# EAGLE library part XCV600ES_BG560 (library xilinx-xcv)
xcv600es_bg560 edit this description Auto generated by make-symbol-device-package-bsdl.ulp Rev. 26 Source: xcv600es_bg560.bsd
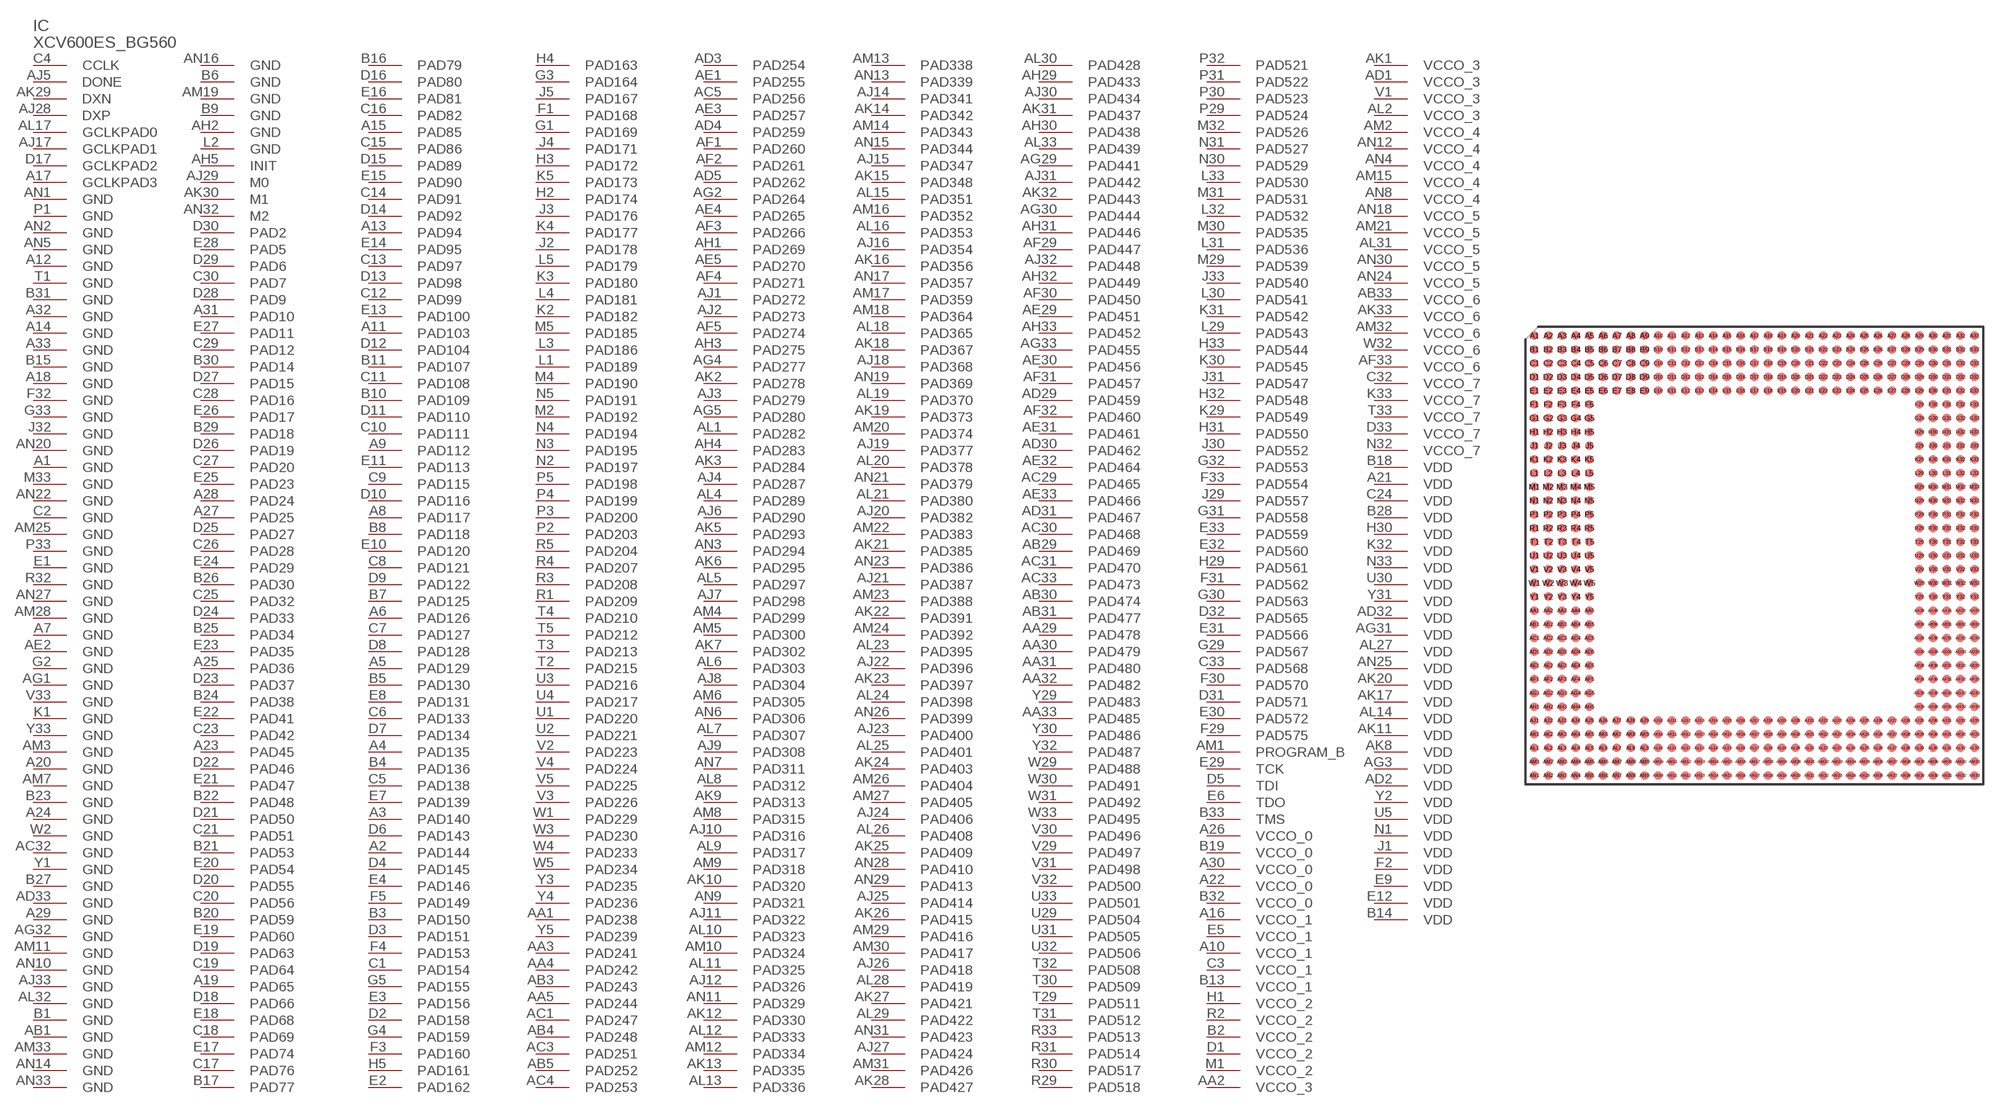
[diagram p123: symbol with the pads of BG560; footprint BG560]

Designator prefix IC

## XCV600ES_BG560 (OC_FARNELL: unknown; OC_NEWARK: unknown)  [BG560]
A1  GND  pwr
A2  PAD144
A3  PAD140
A4  PAD135
A5  PAD129
A6  PAD126
A7  GND  pwr
A8  PAD117
A9  PAD112
A10  VCCO_1  pwr
A11  PAD103
A12  GND  pwr
A13  PAD94
A14  GND  pwr
A15  PAD85
A16  VCCO_1  pwr
A17  GCLKPAD3  in
A18  GND  pwr
A19  PAD65
A20  GND  pwr
A21  VDD  pwr
A22  VCCO_0  pwr
A23  PAD45
A24  GND  pwr
A25  PAD36
A26  VCCO_0  pwr
A27  PAD25
A28  PAD24
A29  GND  pwr
A30  VCCO_0  pwr
A31  PAD10
A32  GND  pwr
A33  GND  pwr
AA1  PAD238
AA2  VCCO_3  pwr
AA3  PAD241
AA4  PAD242
AA5  PAD244
AA29  PAD478
AA30  PAD479
AA31  PAD480
AA32  PAD482
AA33  PAD485
AB1  GND  pwr
AB3  PAD243
AB4  PAD248
AB5  PAD252
AB29  PAD469
AB30  PAD474
AB31  PAD477
AB33  VCCO_6  pwr
AC1  PAD247
AC3  PAD251
AC4  PAD253
AC5  PAD256
AC29  PAD465
AC30  PAD468
AC31  PAD470
AC32  GND  pwr
AC33  PAD473
AD1  VCCO_3  pwr
AD2  VDD  pwr
AD3  PAD254
AD4  PAD259
AD5  PAD262
AD29  PAD459
AD30  PAD462
AD31  PAD467
AD32  VDD  pwr
AD33  GND  pwr
AE1  PAD255
AE2  GND  pwr
AE3  PAD257
AE4  PAD265
AE5  PAD270
AE29  PAD451
AE30  PAD456
AE31  PAD461
AE32  PAD464
AE33  PAD466
AF1  PAD260
AF2  PAD261
AF3  PAD266
AF4  PAD271
AF5  PAD274
AF29  PAD447
AF30  PAD450
AF31  PAD457
AF32  PAD460
AF33  VCCO_6  pwr
AG1  GND  pwr
AG2  PAD264
AG3  VDD  pwr
AG4  PAD277
AG5  PAD280
AG29  PAD441
AG30  PAD444
AG31  VDD  pwr
AG32  GND  pwr
AG33  PAD455
AH1  PAD269
AH2  GND  pwr
AH3  PAD275
AH4  PAD283
AH5  INIT
AH29  PAD433
AH30  PAD438
AH31  PAD446
AH32  PAD449
AH33  PAD452
AJ1  PAD272
AJ2  PAD273
AJ3  PAD279
AJ4  PAD287
AJ5  DONE
AJ6  PAD290
AJ7  PAD298
AJ8  PAD304
AJ9  PAD308
AJ10  PAD316
AJ11  PAD322
AJ12  PAD326
AJ14  PAD341
AJ15  PAD347
AJ16  PAD354
AJ17  GCLKPAD1  in
AJ18  PAD368
AJ19  PAD377
AJ20  PAD382
AJ21  PAD387
AJ22  PAD396
AJ23  PAD400
AJ24  PAD406
AJ25  PAD414
AJ26  PAD418
AJ27  PAD424
AJ28  DXP  pas
AJ29  M0  in
AJ30  PAD434
AJ31  PAD442
AJ32  PAD448
AJ33  GND  pwr
AK1  VCCO_3  pwr
AK2  PAD278
AK3  PAD284
AK5  PAD293
AK6  PAD295
AK7  PAD302
AK8  VDD  pwr
AK9  PAD313
AK10  PAD320
AK11  VDD  pwr
AK12  PAD330
AK13  PAD335
AK14  PAD342
AK15  PAD348
AK16  PAD356
AK17  VDD  pwr
AK18  PAD367
AK19  PAD373
AK20  VDD  pwr
AK21  PAD385
AK22  PAD391
AK23  PAD397
AK24  PAD403
AK25  PAD409
AK26  PAD415
AK27  PAD421
AK28  PAD427
AK29  DXN  pas
AK30  M1  in
AK31  PAD437
AK32  PAD443
AK33  VCCO_6  pwr
AL1  PAD282
AL2  VCCO_3  pwr
AL4  PAD289
AL5  PAD297
AL6  PAD303
AL7  PAD307
AL8  PAD312
AL9  PAD317
AL10  PAD323
AL11  PAD325
AL12  PAD333
AL13  PAD336
AL14  VDD  pwr
AL15  PAD351
AL16  PAD353
AL17  GCLKPAD0  in
AL18  PAD365
AL19  PAD370
AL20  PAD378
AL21  PAD380
AL23  PAD395
AL24  PAD398
AL25  PAD401
AL26  PAD408
AL27  VDD  pwr
AL28  PAD419
AL29  PAD422
AL30  PAD428
AL31  VCCO_5  pwr
AL32  GND  pwr
AL33  PAD439
AM1  PROGRAM_B  in
AM2  VCCO_4  pwr
AM3  GND  pwr
AM4  PAD299
AM5  PAD300
AM6  PAD305
AM7  GND  pwr
AM8  PAD315
AM9  PAD318
AM10  PAD324
AM11  GND  pwr
AM12  PAD334
AM13  PAD338
AM14  PAD343
AM15  VCCO_4  pwr
AM16  PAD352
AM17  PAD359
AM18  PAD364
AM19  GND  pwr
AM20  PAD374
AM21  VCCO_5  pwr
AM22  PAD383
AM23  PAD388
AM24  PAD392
AM25  GND  pwr
AM26  PAD404
AM27  PAD405
AM28  GND  pwr
AM29  PAD416
AM30  PAD417
AM31  PAD426
AM32  VCCO_6  pwr
AM33  GND  pwr
AN1  GND  pwr
AN2  GND  pwr
AN3  PAD294
AN4  VCCO_4  pwr
AN5  GND  pwr
AN6  PAD306
AN7  PAD311
AN8  VCCO_4  pwr
AN9  PAD321
AN10  GND  pwr
AN11  PAD329
AN12  VCCO_4  pwr
AN13  PAD339
AN14  GND  pwr
AN15  PAD344
AN16  GND  pwr
AN17  PAD357
AN18  VCCO_5  pwr
AN19  PAD369
AN20  GND  pwr
AN21  PAD379
AN22  GND  pwr
AN23  PAD386
AN24  VCCO_5  pwr
AN25  VDD  pwr
AN26  PAD399
AN27  GND  pwr
AN28  PAD410
AN29  PAD413
AN30  VCCO_5  pwr
AN31  PAD423
AN32  M2  in
AN33  GND  pwr
B1  GND  pwr
B2  VCCO_2  pwr
B3  PAD150
B4  PAD136
B5  PAD130
B6  GND  pwr
B7  PAD125
B8  PAD118
B9  GND  pwr
B10  PAD109
B11  PAD107
B13  VCCO_1  pwr
B14  VDD  pwr
B15  GND  pwr
B16  PAD79
B17  PAD77
B18  VDD  pwr
B19  VCCO_0  pwr
B20  PAD59
B21  PAD53
B22  PAD48
B23  GND  pwr
B24  PAD38
B25  PAD34
B26  PAD30
B27  GND  pwr
B28  VDD  pwr
B29  PAD18
B30  PAD14
B31  GND  pwr
B32  VCCO_0  pwr
B33  TMS  in
C1  PAD154
C2  GND  pwr
C3  VCCO_1  pwr
C4  CCLK
C5  PAD138
C6  PAD133
C7  PAD127
C8  PAD121
C9  PAD115
C10  PAD111
C11  PAD108
C12  PAD99
C13  PAD97
C14  PAD91
C15  PAD86
C16  PAD82
C17  PAD76
C18  PAD69
C19  PAD64
C20  PAD56
C21  PAD51
C23  PAD42
C24  VDD  pwr
C25  PAD32
C26  PAD28
C27  PAD20
C28  PAD16
C29  PAD12
C30  PAD7
C32  VCCO_7  pwr
C33  PAD568
D1  VCCO_2  pwr
D2  PAD158
D3  PAD151
D4  PAD145
D5  TDI  in
D6  PAD143
D7  PAD134
D8  PAD128
D9  PAD122
D10  PAD116
D11  PAD110
D12  PAD104
D13  PAD98
D14  PAD92
D15  PAD89
D16  PAD80
D17  GCLKPAD2  in
D18  PAD66
D19  PAD63
D20  PAD55
D21  PAD50
D22  PAD46
D23  PAD37
D24  PAD33
D25  PAD27
D26  PAD19
D27  PAD15
D28  PAD9
D29  PAD6
D30  PAD2
D31  PAD571
D32  PAD565
D33  VCCO_7  pwr
E1  GND  pwr
E2  PAD162
E3  PAD156
E4  PAD146
E5  VCCO_1  pwr
E6  TDO  out
E7  PAD139
E8  PAD131
E9  VDD  pwr
E10  PAD120
E11  PAD113
E12  VDD  pwr
E13  PAD100
E14  PAD95
E15  PAD90
E16  PAD81
E17  PAD74
E18  PAD68
E19  PAD60
E20  PAD54
E21  PAD47
E22  PAD41
E23  PAD35
E24  PAD29
E25  PAD23
E26  PAD17
E27  PAD11
E28  PAD5
E29  TCK  in
E30  PAD572
E31  PAD566
E32  PAD560
E33  PAD559
F1  PAD168
F2  VDD  pwr
F3  PAD160
F4  PAD153
F5  PAD149
F29  PAD575
F30  PAD570
F31  PAD562
F32  GND  pwr
F33  PAD554
G1  PAD169
G2  GND  pwr
G3  PAD164
G4  PAD159
G5  PAD155
G29  PAD567
G30  PAD563
G31  PAD558
G32  PAD553
G33  GND  pwr
H1  VCCO_2  pwr
H2  PAD174
H3  PAD172
H4  PAD163
H5  PAD161
H29  PAD561
H30  VDD  pwr
H31  PAD550
H32  PAD548
H33  PAD544
J1  VDD  pwr
J2  PAD178
J3  PAD176
J4  PAD171
J5  PAD167
J29  PAD557
J30  PAD552
J31  PAD547
J32  GND  pwr
J33  PAD540
K1  GND  pwr
K2  PAD182
K3  PAD180
K4  PAD177
K5  PAD173
K29  PAD549
K30  PAD545
K31  PAD542
K32  VDD  pwr
K33  VCCO_7  pwr
L1  PAD189
L2  GND  pwr
L3  PAD186
L4  PAD181
L5  PAD179
L29  PAD543
L30  PAD541
L31  PAD536
L32  PAD532
L33  PAD530
M1  VCCO_2  pwr
M2  PAD192
M4  PAD190
M5  PAD185
M29  PAD539
M30  PAD535
M31  PAD531
M32  PAD526
M33  GND  pwr
N1  VDD  pwr
N2  PAD197
N3  PAD195
N4  PAD194
N5  PAD191
N30  PAD529
N31  PAD527
N32  VCCO_7  pwr
N33  VDD  pwr
P1  GND  pwr
P2  PAD203
P3  PAD200
P4  PAD199
P5  PAD198
P29  PAD524
P30  PAD523
P31  PAD522
P32  PAD521
P33  GND  pwr
R1  PAD209
R2  VCCO_2  pwr
R3  PAD208
R4  PAD207
R5  PAD204
R29  PAD518
R30  PAD517
R31  PAD514
R32  GND  pwr
R33  PAD513
T1  GND  pwr
T2  PAD215
T3  PAD213
T4  PAD210
T5  PAD212
T29  PAD511
T30  PAD509
T31  PAD512
T32  PAD508
T33  VCCO_7  pwr
U1  PAD220
U2  PAD221
U3  PAD216
U4  PAD217
U5  VDD  pwr
U29  PAD504
U30  VDD  pwr
U31  PAD505
U32  PAD506
U33  PAD501
V1  VCCO_3  pwr
V2  PAD223
V3  PAD226
V4  PAD224
V5  PAD225
V29  PAD497
V30  PAD496
V31  PAD498
V32  PAD500
V33  GND  pwr
W1  PAD229
W2  GND  pwr
W3  PAD230
W4  PAD233
W5  PAD234
W29  PAD488
W30  PAD491
W31  PAD492
W32  VCCO_6  pwr
W33  PAD495
Y1  GND  pwr
Y2  VDD  pwr
Y3  PAD235
Y4  PAD236
Y5  PAD239
Y29  PAD483
Y30  PAD486
Y31  VDD  pwr
Y32  PAD487
Y33  GND  pwr

## Footprint BG560 (pad centres in mm)
Metal BGA (BG560) Auto generated by make-symbol-device-package-bsdl.ulp Rev. 26 Source: xcv1000_bg560_1532.bsd; bg560.pdf
smd 0.8 x 0.8: A1 -20.32,20.32; A2 -19.05,20.32; A3 -17.78,20.32; A4 -16.51,20.32; A5 -15.24,20.32; A6 -13.97,20.32; A7 -12.7,20.32; A8 -11.43,20.32; A9 -10.16,20.32; A10 -8.89,20.32; A11 -7.62,20.32; A12 -6.35,20.32; A13 -5.08,20.32; A14 -3.81,20.32; A15 -2.54,20.32; A16 -1.27,20.32; A17 0,20.32; A18 1.27,20.32; A19 2.54,20.32; A20 3.81,20.32; A21 5.08,20.32; A22 6.35,20.32; A23 7.62,20.32; A24 8.89,20.32; A25 10.16,20.32; A26 11.43,20.32; A27 12.7,20.32; A28 13.97,20.32; A29 15.24,20.32; A30 16.51,20.32; A31 17.78,20.32; A32 19.05,20.32; A33 20.32,20.32; AA1 -20.32,-5.08; AA2 -19.05,-5.08; AA3 -17.78,-5.08; AA4 -16.51,-5.08; AA5 -15.24,-5.08; AA29 15.24,-5.08; AA30 16.51,-5.08; AA31 17.78,-5.08; AA32 19.05,-5.08; AA33 20.32,-5.08; AB1 -20.32,-6.35; AB2 -19.05,-6.35; AB3 -17.78,-6.35; AB4 -16.51,-6.35; AB5 -15.24,-6.35; AB29 15.24,-6.35; AB30 16.51,-6.35; AB31 17.78,-6.35; AB32 19.05,-6.35; AB33 20.32,-6.35; AC1 -20.32,-7.62; AC2 -19.05,-7.62; AC3 -17.78,-7.62; AC4 -16.51,-7.62; AC5 -15.24,-7.62; AC29 15.24,-7.62; AC30 16.51,-7.62; AC31 17.78,-7.62; AC32 19.05,-7.62; AC33 20.32,-7.62; AD1 -20.32,-8.89; AD2 -19.05,-8.89; AD3 -17.78,-8.89; AD4 -16.51,-8.89; AD5 -15.24,-8.89; AD29 15.24,-8.89; AD30 16.51,-8.89; AD31 17.78,-8.89; AD32 19.05,-8.89; AD33 20.32,-8.89; AE1 -20.32,-10.16; AE2 -19.05,-10.16; AE3 -17.78,-10.16; AE4 -16.51,-10.16; AE5 -15.24,-10.16; AE29 15.24,-10.16; AE30 16.51,-10.16; AE31 17.78,-10.16; AE32 19.05,-10.16; AE33 20.32,-10.16; AF1 -20.32,-11.43; AF2 -19.05,-11.43; AF3 -17.78,-11.43; AF4 -16.51,-11.43; AF5 -15.24,-11.43; AF29 15.24,-11.43; AF30 16.51,-11.43; AF31 17.78,-11.43; AF32 19.05,-11.43; AF33 20.32,-11.43; AG1 -20.32,-12.7; AG2 -19.05,-12.7; AG3 -17.78,-12.7; AG4 -16.51,-12.7; AG5 -15.24,-12.7; AG29 15.24,-12.7; AG30 16.51,-12.7; AG31 17.78,-12.7; AG32 19.05,-12.7; AG33 20.32,-12.7; AH1 -20.32,-13.97; AH2 -19.05,-13.97; AH3 -17.78,-13.97; AH4 -16.51,-13.97; AH5 -15.24,-13.97; AH29 15.24,-13.97; AH30 16.51,-13.97; AH31 17.78,-13.97; AH32 19.05,-13.97; AH33 20.32,-13.97; AJ1 -20.32,-15.24; AJ2 -19.05,-15.24; AJ3 -17.78,-15.24; AJ4 -16.51,-15.24; AJ5 -15.24,-15.24; AJ6 -13.97,-15.24; AJ7 -12.7,-15.24; AJ8 -11.43,-15.24; AJ9 -10.16,-15.24; AJ10 -8.89,-15.24; AJ11 -7.62,-15.24; AJ12 -6.35,-15.24; AJ13 -5.08,-15.24; AJ14 -3.81,-15.24; AJ15 -2.54,-15.24; AJ16 -1.27,-15.24; AJ17 0,-15.24; AJ18 1.27,-15.24; AJ19 2.54,-15.24; AJ20 3.81,-15.24; AJ21 5.08,-15.24; AJ22 6.35,-15.24; AJ23 7.62,-15.24; AJ24 8.89,-15.24; AJ25 10.16,-15.24; AJ26 11.43,-15.24; AJ27 12.7,-15.24; AJ28 13.97,-15.24; AJ29 15.24,-15.24; AJ30 16.51,-15.24; AJ31 17.78,-15.24; AJ32 19.05,-15.24; AJ33 20.32,-15.24; AK1 -20.32,-16.51; AK2 -19.05,-16.51; AK3 -17.78,-16.51; AK4 -16.51,-16.51; AK5 -15.24,-16.51; AK6 -13.97,-16.51; AK7 -12.7,-16.51; AK8 -11.43,-16.51; AK9 -10.16,-16.51; AK10 -8.89,-16.51; AK11 -7.62,-16.51; AK12 -6.35,-16.51; AK13 -5.08,-16.51; AK14 -3.81,-16.51; AK15 -2.54,-16.51; AK16 -1.27,-16.51; AK17 0,-16.51; AK18 1.27,-16.51; AK19 2.54,-16.51; AK20 3.81,-16.51; AK21 5.08,-16.51; AK22 6.35,-16.51; AK23 7.62,-16.51; AK24 8.89,-16.51; AK25 10.16,-16.51; AK26 11.43,-16.51; AK27 12.7,-16.51; AK28 13.97,-16.51; AK29 15.24,-16.51; AK30 16.51,-16.51; AK31 17.78,-16.51; AK32 19.05,-16.51; AK33 20.32,-16.51; AL1 -20.32,-17.78; AL2 -19.05,-17.78; AL3 -17.78,-17.78; AL4 -16.51,-17.78; AL5 -15.24,-17.78; AL6 -13.97,-17.78; AL7 -12.7,-17.78; AL8 -11.43,-17.78; AL9 -10.16,-17.78; AL10 -8.89,-17.78; AL11 -7.62,-17.78; AL12 -6.35,-17.78; AL13 -5.08,-17.78; AL14 -3.81,-17.78; AL15 -2.54,-17.78; AL16 -1.27,-17.78; AL17 0,-17.78; AL18 1.27,-17.78; AL19 2.54,-17.78; AL20 3.81,-17.78; AL21 5.08,-17.78; AL22 6.35,-17.78; AL23 7.62,-17.78; AL24 8.89,-17.78; AL25 10.16,-17.78; AL26 11.43,-17.78; AL27 12.7,-17.78; AL28 13.97,-17.78; AL29 15.24,-17.78; AL30 16.51,-17.78; AL31 17.78,-17.78; AL32 19.05,-17.78; AL33 20.32,-17.78; AM1 -20.32,-19.05; AM2 -19.05,-19.05; AM3 -17.78,-19.05; AM4 -16.51,-19.05; AM5 -15.24,-19.05; AM6 -13.97,-19.05; AM7 -12.7,-19.05; AM8 -11.43,-19.05; AM9 -10.16,-19.05; AM10 -8.89,-19.05; AM11 -7.62,-19.05; AM12 -6.35,-19.05; AM13 -5.08,-19.05; AM14 -3.81,-19.05; AM15 -2.54,-19.05; AM16 -1.27,-19.05; AM17 0,-19.05; AM18 1.27,-19.05; AM19 2.54,-19.05; AM20 3.81,-19.05; AM21 5.08,-19.05; AM22 6.35,-19.05; AM23 7.62,-19.05; AM24 8.89,-19.05; AM25 10.16,-19.05; AM26 11.43,-19.05; AM27 12.7,-19.05; AM28 13.97,-19.05; AM29 15.24,-19.05; AM30 16.51,-19.05; AM31 17.78,-19.05; AM32 19.05,-19.05; AM33 20.32,-19.05; AN1 -20.32,-20.32; AN2 -19.05,-20.32; AN3 -17.78,-20.32; AN4 -16.51,-20.32; AN5 -15.24,-20.32; AN6 -13.97,-20.32; AN7 -12.7,-20.32; AN8 -11.43,-20.32; AN9 -10.16,-20.32; AN10 -8.89,-20.32; AN11 -7.62,-20.32; AN12 -6.35,-20.32; AN13 -5.08,-20.32; AN14 -3.81,-20.32; AN15 -2.54,-20.32; AN16 -1.27,-20.32; AN17 0,-20.32; AN18 1.27,-20.32; AN19 2.54,-20.32; AN20 3.81,-20.32; AN21 5.08,-20.32; AN22 6.35,-20.32; AN23 7.62,-20.32; AN24 8.89,-20.32; AN25 10.16,-20.32; AN26 11.43,-20.32; AN27 12.7,-20.32; AN28 13.97,-20.32; AN29 15.24,-20.32; AN30 16.51,-20.32; AN31 17.78,-20.32; AN32 19.05,-20.32; AN33 20.32,-20.32; B1 -20.32,19.05; B2 -19.05,19.05; B3 -17.78,19.05; B4 -16.51,19.05; B5 -15.24,19.05; B6 -13.97,19.05; B7 -12.7,19.05; B8 -11.43,19.05; B9 -10.16,19.05; B10 -8.89,19.05; B11 -7.62,19.05; B12 -6.35,19.05; B13 -5.08,19.05; B14 -3.81,19.05; B15 -2.54,19.05; B16 -1.27,19.05; B17 0,19.05; B18 1.27,19.05; B19 2.54,19.05; B20 3.81,19.05; B21 5.08,19.05; B22 6.35,19.05; B23 7.62,19.05; B24 8.89,19.05; B25 10.16,19.05; B26 11.43,19.05; B27 12.7,19.05; B28 13.97,19.05; B29 15.24,19.05; B30 16.51,19.05; B31 17.78,19.05; B32 19.05,19.05; B33 20.32,19.05; C1 -20.32,17.78; C2 -19.05,17.78; C3 -17.78,17.78; C4 -16.51,17.78; C5 -15.24,17.78; C6 -13.97,17.78; C7 -12.7,17.78; C8 -11.43,17.78; C9 -10.16,17.78; C10 -8.89,17.78; C11 -7.62,17.78; C12 -6.35,17.78; C13 -5.08,17.78; C14 -3.81,17.78; C15 -2.54,17.78; C16 -1.27,17.78; C17 0,17.78; C18 1.27,17.78; C19 2.54,17.78; C20 3.81,17.78; C21 5.08,17.78; C22 6.35,17.78; C23 7.62,17.78; C24 8.89,17.78; C25 10.16,17.78; C26 11.43,17.78; C27 12.7,17.78; C28 13.97,17.78; C29 15.24,17.78; C30 16.51,17.78; C31 17.78,17.78; C32 19.05,17.78; C33 20.32,17.78; D1 -20.32,16.51; D2 -19.05,16.51; D3 -17.78,16.51; D4 -16.51,16.51; D5 -15.24,16.51; D6 -13.97,16.51; D7 -12.7,16.51; D8 -11.43,16.51; D9 -10.16,16.51; D10 -8.89,16.51; D11 -7.62,16.51; D12 -6.35,16.51; D13 -5.08,16.51; D14 -3.81,16.51; D15 -2.54,16.51; D16 -1.27,16.51; D17 0,16.51; D18 1.27,16.51; D19 2.54,16.51; D20 3.81,16.51; D21 5.08,16.51; D22 6.35,16.51; D23 7.62,16.51; D24 8.89,16.51; D25 10.16,16.51; D26 11.43,16.51; D27 12.7,16.51; D28 13.97,16.51; D29 15.24,16.51; D30 16.51,16.51; D31 17.78,16.51; D32 19.05,16.51; D33 20.32,16.51; E1 -20.32,15.24; E2 -19.05,15.24; E3 -17.78,15.24; E4 -16.51,15.24; E5 -15.24,15.24; E6 -13.97,15.24; E7 -12.7,15.24; E8 -11.43,15.24; E9 -10.16,15.24; E10 -8.89,15.24; E11 -7.62,15.24; E12 -6.35,15.24; E13 -5.08,15.24; E14 -3.81,15.24; E15 -2.54,15.24; E16 -1.27,15.24; E17 0,15.24; E18 1.27,15.24; E19 2.54,15.24; E20 3.81,15.24; E21 5.08,15.24; E22 6.35,15.24; E23 7.62,15.24; E24 8.89,15.24; E25 10.16,15.24; E26 11.43,15.24; E27 12.7,15.24; E28 13.97,15.24; E29 15.24,15.24; E30 16.51,15.24; E31 17.78,15.24; E32 19.05,15.24; E33 20.32,15.24; F1 -20.32,13.97; F2 -19.05,13.97; F3 -17.78,13.97; F4 -16.51,13.97; F5 -15.24,13.97; F29 15.24,13.97; F30 16.51,13.97; F31 17.78,13.97; F32 19.05,13.97; F33 20.32,13.97; G1 -20.32,12.7; G2 -19.05,12.7; G3 -17.78,12.7; G4 -16.51,12.7; G5 -15.24,12.7; G29 15.24,12.7; G30 16.51,12.7; G31 17.78,12.7; G32 19.05,12.7; G33 20.32,12.7; H1 -20.32,11.43; H2 -19.05,11.43; H3 -17.78,11.43; H4 -16.51,11.43; H5 -15.24,11.43; H29 15.24,11.43; H30 16.51,11.43; H31 17.78,11.43; H32 19.05,11.43; H33 20.32,11.43; J1 -20.32,10.16; J2 -19.05,10.16; J3 -17.78,10.16; J4 -16.51,10.16; J5 -15.24,10.16; J29 15.24,10.16; J30 16.51,10.16; J31 17.78,10.16; J32 19.05,10.16; J33 20.32,10.16; K1 -20.32,8.89; K2 -19.05,8.89; K3 -17.78,8.89; K4 -16.51,8.89; K5 -15.24,8.89; K29 15.24,8.89; K30 16.51,8.89; K31 17.78,8.89; K32 19.05,8.89; K33 20.32,8.89; L1 -20.32,7.62; L2 -19.05,7.62; L3 -17.78,7.62; L4 -16.51,7.62; L5 -15.24,7.62; L29 15.24,7.62; L30 16.51,7.62; L31 17.78,7.62; L32 19.05,7.62; L33 20.32,7.62; M1 -20.32,6.35; M2 -19.05,6.35; M3 -17.78,6.35; M4 -16.51,6.35; M5 -15.24,6.35; M29 15.24,6.35; M30 16.51,6.35; M31 17.78,6.35; M32 19.05,6.35; M33 20.32,6.35; N1 -20.32,5.08; N2 -19.05,5.08; N3 -17.78,5.08; N4 -16.51,5.08; N5 -15.24,5.08; N29 15.24,5.08; N30 16.51,5.08; N31 17.78,5.08; N32 19.05,5.08; N33 20.32,5.08; P1 -20.32,3.81; P2 -19.05,3.81; P3 -17.78,3.81; P4 -16.51,3.81; P5 -15.24,3.81; P29 15.24,3.81; P30 16.51,3.81; P31 17.78,3.81; P32 19.05,3.81; P33 20.32,3.81; R1 -20.32,2.54; R2 -19.05,2.54; R3 -17.78,2.54; R4 -16.51,2.54; R5 -15.24,2.54; R29 15.24,2.54; R30 16.51,2.54; R31 17.78,2.54; R32 19.05,2.54; R33 20.32,2.54; T1 -20.32,1.27; T2 -19.05,1.27; T3 -17.78,1.27; T4 -16.51,1.27; T5 -15.24,1.27; T29 15.24,1.27; T30 16.51,1.27; T31 17.78,1.27; T32 19.05,1.27; T33 20.32,1.27; U1 -20.32,0; U2 -19.05,0; U3 -17.78,0; U4 -16.51,0; U5 -15.24,0; U29 15.24,0; U30 16.51,0; U31 17.78,0; U32 19.05,0; U33 20.32,0; V1 -20.32,-1.27; V2 -19.05,-1.27; V3 -17.78,-1.27; V4 -16.51,-1.27; V5 -15.24,-1.27; V29 15.24,-1.27; V30 16.51,-1.27; V31 17.78,-1.27; V32 19.05,-1.27; V33 20.32,-1.27; W1 -20.32,-2.54; W2 -19.05,-2.54; W3 -17.78,-2.54; W4 -16.51,-2.54; W5 -15.24,-2.54; W29 15.24,-2.54; W30 16.51,-2.54; W31 17.78,-2.54; W32 19.05,-2.54; W33 20.32,-2.54; Y1 -20.32,-3.81; Y2 -19.05,-3.81; Y3 -17.78,-3.81; Y4 -16.51,-3.81; Y5 -15.24,-3.81; Y29 15.24,-3.81; Y30 16.51,-3.81; Y31 17.78,-3.81; Y32 19.05,-3.81; Y33 20.32,-3.81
